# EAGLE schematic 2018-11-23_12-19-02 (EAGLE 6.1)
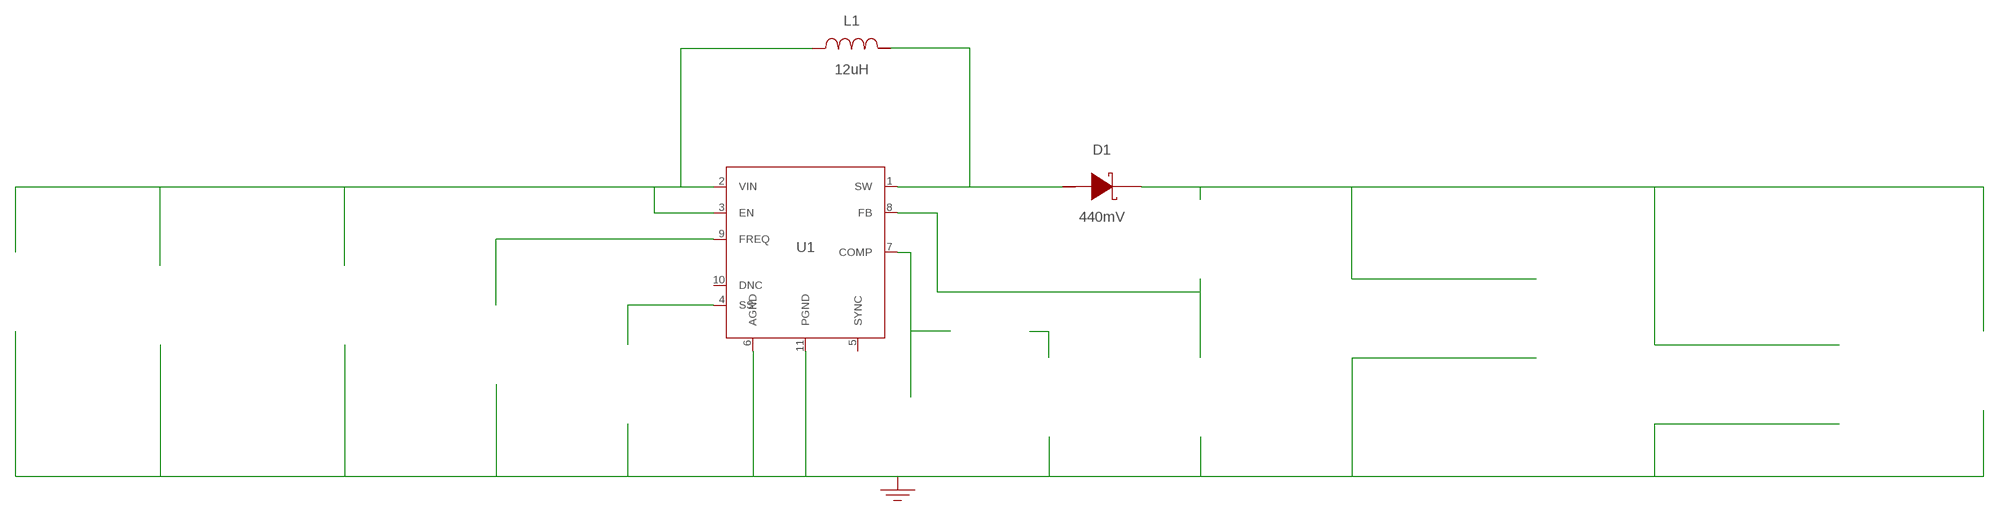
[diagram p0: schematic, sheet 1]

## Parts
CCOMP  68nF  C3216C0G1H683J160AAC3216C0G1H683J160AA  [1206]  (not placed on a sheet)
CCOMP2  1.1nF  C0402C112J5GAC7867C0402C112J5GAC7867  [0402]  (not placed on a sheet)
CIN  10uF  C2012X5R1V106K085ACC2012X5R1V106K085AC  [0805]  (not placed on a sheet)
CINX  100nF  UMK212B7104KG-TUMK212B7104KG-T  [0805]  (not placed on a sheet)
COUT  6.8uF  C3216X5R1H685K160ABC3216X5R1H685K160AB  [1206_180]  (not placed on a sheet)
COUT_2  6.8uF  C3216X5R1H685K160ABC3216X5R1H685K160AB  [1206_180]  (not placed on a sheet)
COUT_3  6.8uF  C3216X5R1H685K160ABC3216X5R1H685K160AB  [1206_180]  (not placed on a sheet)
COUTX  1uF  C1608X5R1H105K080ABC1608X5R1H105K080AB  [0603]  (not placed on a sheet)
COUTX_2  1uF  C1608X5R1H105K080ABC1608X5R1H105K080AB  [0603]  (not placed on a sheet)
COUTX_3  1uF  C1608X5R1H105K080ABC1608X5R1H105K080AB  [0603]  (not placed on a sheet)
CSS  22nF  GRM188R71C223KA01DGRM188R71C223KA01D  [0603]  (not placed on a sheet)
D1  440mV  SL44-E3/57TSL44-E3/57T  [SMC]
GND  WB_GND  WB_GNDWB_GND  [WB_GND]
IOUT  WB_CURRENT_LOAD  WB_CURRENT_LOADWB_CURRENT_LOAD  [WB_CURRENT_LOAD]  (not placed on a sheet)
L1  12uH  MSS1260-123MLBMSS1260-123MLB  [MSS1260]
RCOMP  1.96k  ERJ-6ENF1961VERJ-6ENF1961V  [0805]  (not placed on a sheet)
RFBB  10k  CRCW080510K0FKEACRCW080510K0FKEA  [0805]  (not placed on a sheet)
RFBT  232k  ERJ-6ENF2323VERJ-6ENF2323V  [0805]  (not placed on a sheet)
RT  32.4k  ERJ-6ENF3242VERJ-6ENF3242V  [0805]  (not placed on a sheet)
U1  TPS55340QRTERQ1  TPS55340QRTERQ1TPS55340QRTERQ1  [S-PWQFN-N16]
VIN  WB_BATTERY  WB_BATTERYWB_BATTERY  [WB_BATTERY]  (not placed on a sheet)

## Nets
0: Ccomp2.1@1 Ccomp.2@2 Cin.2@2 Cinx.2@2 Cout.2@2 Cout_2.2@2 Cout_3.2@2 Coutx.2@2 Coutx_2.2@2 Coutx_3.2@2 Css.2@2 GND.1 Iout.-@2 Rfbb.2@2 Rt.2@2 U1.6(AGND) U1.11(PGND) U1.12(PGND) U1.13(PGND) U1.17(ETPAD) Vin.-@2
2: Cout.1@1 Cout_2.1@1 Cout_3.1@1 Coutx.1@1 Coutx_2.1@1 Coutx_3.1@1 D1.1(K) Iout.+@1 Rfbt.1@1
3: Cin.1@1 Cinx.1@1 L1.1 U1.2(VIN) U1.3(EN) Vin.+@1
4: Css.1@1 U1.4(SS)
5: Rfbb.1@1 Rfbt.2@2 U1.8(FB)
6: Ccomp2.2@2 Rcomp.2@2 U1.7(COMP)
7: D1.2(A) L1.2 U1.1(SW) U1.15(SW) U1.16(SW)
8: Rt.1@1 U1.9(FREQ)
10: Ccomp.1@1 Rcomp.1@1
Unconnected: CCOMP2.1 CCOMP2.2 CCOMP.1 CCOMP.2 CIN.1 CIN.2 CINX.1 CINX.2 COUT.1 COUT.2 COUT_2.1 COUT_2.2 COUT_3.1 COUT_3.2 COUTX.1 COUTX.2 COUTX_2.1 COUTX_2.2 COUTX_3.1 COUTX_3.2 CSS.1 CSS.2 IOUT.1(+) IOUT.2(-) RCOMP.1 RCOMP.2 RFBB.1 RFBB.2 RFBT.1 RFBT.2 RT.1 RT.2 U1.5(SYNC) U1.10(DNC) U1.14(DNC) VIN.1(+) VIN.2(-)

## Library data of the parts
CCOMP = AcceleratedDesigns_Lib:C3216C0G1H683J160AA; Cap: 6.8E-8; Datasheet_URL: http://product.tdk.com/capacitor/mlcc/en/documents/mlcc%5Fcommercial%5Fgeneral%5Fen.pdf; ESR: 0.0; IRMS: 0.0; Manufacturer_Name: TDK; Manufacturer_Part_Number: C3216C0G1H683J160AA; VDC: 5.0; Vendor: TDK
CCOMP2 = AcceleratedDesigns_Lib:C0402C112J5GAC7867; Cap: 1.1E-9; Datasheet_URL: http://www.kemet.com/docfinder?Partnumber%3DC0402C112J5GAC7867; ESR: 0.0; IRMS: 0.0; Manufacturer_Name: Kemet; Manufacturer_Part_Number: C0402C112J5GAC7867; VDC: 5.0; Vendor: Kemet
CIN = AcceleratedDesigns_Lib:C2012X5R1V106K085AC; Cap: 1.0E-5; Datasheet_URL: https://product.tdk.com/en/search/capacitor/ceramic/mlcc/info?part%5Fno%3DC2012X5R1V106K085AC; ESR: 0.002818; IRMS: 3.88676; Manufacturer_Name: TDK; Manufacturer_Part_Number: C2012X5R1V106K085AC; VDC: 35.0; Vendor: TDK
CINX = AcceleratedDesigns_Lib:UMK212B7104KG-T; Cap: 1.0E-7; ESR: 0.0; IRMS: 0.0; Manufacturer_Name: Taiyo Yuden; Manufacturer_Part_Number: UMK212B7104KG-T; VDC: 50.0; Vendor: Taiyo Yuden
COUT COUT_2 COUT_3 = AcceleratedDesigns_Lib:C3216X5R1H685K160AB; Cap: 6.8E-6; Datasheet_URL: https://product.tdk.com/en/search/capacitor/ceramic/mlcc/info?part%5Fno%3DC3216X5R1H685K160AB; ESR: 0.003202; IRMS: 4.05527; Manufacturer_Name: TDK; Manufacturer_Part_Number: C3216X5R1H685K160AB; VDC: 50.0; Vendor: TDK
COUTX COUTX_2 COUTX_3 = AcceleratedDesigns_Lib:C1608X5R1H105K080AB; Cap: 1.0E-6; Datasheet_URL: https://product.tdk.com/en/search/capacitor/ceramic/mlcc/info?part%5Fno%3DC1608X5R1H105K080AB; ESR: 0.005522; IRMS: 2.21617; Manufacturer_Name: TDK; Manufacturer_Part_Number: C1608X5R1H105K080AB; VDC: 50.0; Vendor: TDK
CSS = AcceleratedDesigns_Lib:GRM188R71C223KA01D; Cap: 2.2E-8; ESR: 0.0; IRMS: 0.0; Manufacturer_Name: MuRata; Manufacturer_Part_Number: GRM188R71C223KA01D; VDC: 16.0; Vendor: MuRata
D1 = AcceleratedDesigns_Lib:SL44-E3/57T; Datasheet_URL: http://www.vishay.com/docs/88742/88742.pdf; Io: 4.0; Manufacturer_Name: Vishay-Semiconductor; Manufacturer_Part_Number: SL44-E3/57T; VFatIo: 0.44; VRRM: 40.0; Vendor: Vishay-Semiconductor
GND = AcceleratedDesigns_Lib:WB_GND; Manufacturer_Name: WB_GND; Manufacturer_Part_Number: WB_GND; PowerPortType: POWER_GROUND; Value: Value
IOUT = AcceleratedDesigns_Lib:WB_CURRENT_LOAD; Manufacturer_Name: WB_CURRENT_LOAD; Manufacturer_Part_Number: WB_CURRENT_LOAD; PowerPortType: POWER_GROUND; Value: Value
L1 = AcceleratedDesigns_Lib:MSS1260-123MLB; DCR: 0.02; IDC: 3.7; L: 1.2E-5; Manufacturer_Name: Coilcraft; Manufacturer_Part_Number: MSS1260-123MLB; Vendor: Coilcraft
RCOMP = AcceleratedDesigns_Lib:ERJ-6ENF1961V; Manufacturer_Name: Panasonic; Manufacturer_Part_Number: ERJ-6ENF1961V; Power: 0.125; Resistance: 1960.0; Tolerance: 1.0; Vendor: Panasonic
RFBB = AcceleratedDesigns_Lib:CRCW080510K0FKEA; Manufacturer_Name: Vishay-Dale; Manufacturer_Part_Number: CRCW080510K0FKEA; Power: 0.125; Resistance: 10000.0; Tolerance: 1.0; Vendor: Vishay-Dale
RFBT = AcceleratedDesigns_Lib:ERJ-6ENF2323V; Manufacturer_Name: Panasonic; Manufacturer_Part_Number: ERJ-6ENF2323V; Power: 0.125; Resistance: 232000.0; Tolerance: 1.0; Vendor: Panasonic
RT = AcceleratedDesigns_Lib:ERJ-6ENF3242V; Manufacturer_Name: Panasonic; Manufacturer_Part_Number: ERJ-6ENF3242V; Power: 0.125; Resistance: 32400.0; Tolerance: 1.0; Vendor: Panasonic
U1 = AcceleratedDesigns_Lib:TPS55340QRTERQ1; Datasheet_URL: http://www.ti.com/product/tps55340; Frequency: 1200000.0; Imax: 5.0; Manufacturer_Name: Texas Instruments; Manufacturer_Part_Number: TPS55340RTER; Mktg_Package: HTSSOP; Package: HTSSOP; Vendor: Texas Instruments
VIN = AcceleratedDesigns_Lib:WB_BATTERY; Manufacturer_Name: WB_BATTERY; Manufacturer_Part_Number: WB_BATTERY; PowerPortType: POWER_GROUND; Value: Value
